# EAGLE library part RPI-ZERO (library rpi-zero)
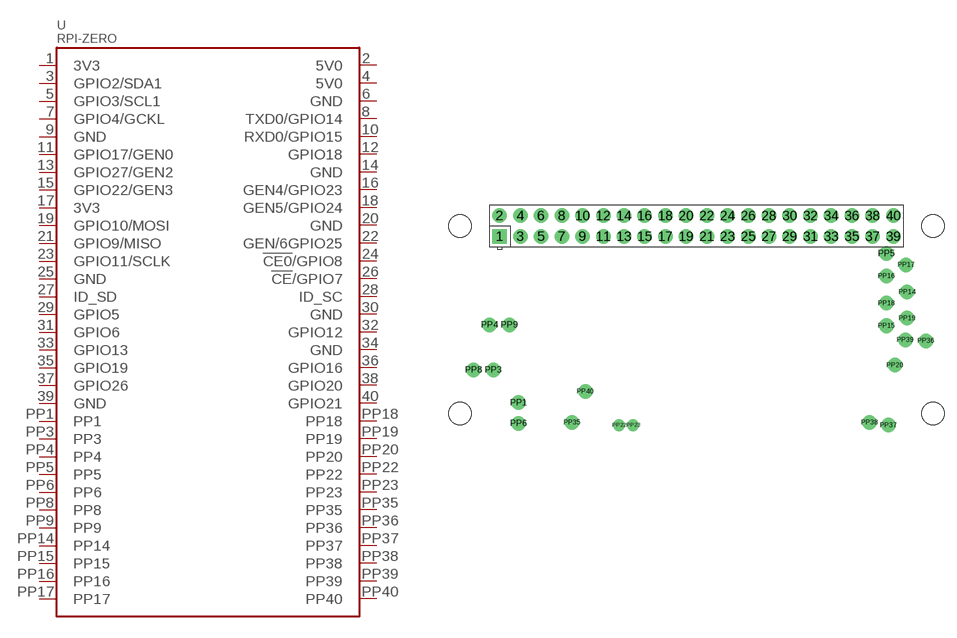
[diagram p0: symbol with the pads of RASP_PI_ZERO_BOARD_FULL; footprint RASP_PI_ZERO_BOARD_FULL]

Designator prefix -

## RPI-ZERO  [RASP_PI_ZERO_BOARD_FULL]
1  3V3  sup
2  5V0  sup
3  GPIO2/SDA1
4  5V0  sup
5  GPIO3/SCL1
6  GND  sup
7  GPIO4/GCKL
8  TXD0/GPIO14
9  GND  sup
10  RXD0/GPIO15
11  GPIO17/GEN0
12  GPIO18
13  GPIO27/GEN2
14  GND  sup
15  GPIO22/GEN3
16  GEN4/GPIO23
17  3V3  sup
18  GEN5/GPIO24
19  GPIO10/MOSI
20  GND  sup
21  GPIO9/MISO
22  GEN/6GPIO25
23  GPIO11/SCLK
24  !CE0!/GPIO8
25  GND  sup
26  !CE!/GPIO7
27  ID_SD
28  ID_SC
29  GPIO5
30  GND  sup
31  GPIO6
32  GPIO12
33  GPIO13
34  GND  sup
35  GPIO19
36  GPIO16
37  GPIO26
38  GPIO20
39  GND  sup
40  GPIO21
PP1  PP1
PP3  PP3
PP4  PP4
PP5  PP5
PP6  PP6
PP8  PP8
PP9  PP9
PP14  PP14
PP15  PP15
PP16  PP16
PP17  PP17
PP18  PP18
PP19  PP19
PP20  PP20  oc
PP22  PP22
PP23  PP23
PP35  PP35
PP36  PP36
PP37  PP37
PP38  PP38
PP39  PP39
PP40  PP40

## Footprint RASP_PI_ZERO_BOARD_FULL (pad centres in mm)
Raspberry Pi board model B+, full outline with position of big connectors & drill holes
drill 1 pad 1.778 square: 1 8.37,25.23
drill 1 pad 1.778: 2 8.37,27.77; 3 10.91,25.23; 4 10.91,27.77; 5 13.45,25.23; 6 13.45,27.77; 7 15.99,25.23; 8 15.99,27.77; 9 18.53,25.23; 10 18.53,27.77; 11 21.07,25.23; 12 21.07,27.77; 13 23.61,25.23; 14 23.61,27.77; 15 26.15,25.23; 16 26.15,27.77; 17 28.69,25.23; 18 28.69,27.77; 19 31.23,25.23; 20 31.23,27.77; 21 33.77,25.23; 22 33.77,27.77; 23 36.31,25.23; 24 36.31,27.77; 25 38.85,25.23; 26 38.85,27.77; 27 41.39,25.23; 28 41.39,27.77; 29 43.93,25.23; 30 43.93,27.77; 31 46.47,25.23; 32 46.47,27.77; 33 49.01,25.23; 34 49.01,27.77; 35 51.55,25.23; 36 51.55,27.77; 37 54.09,25.23; 38 54.09,27.77; 39 56.63,25.23; 40 56.63,27.77
drill 0.8 pad 1.778: PP1 10.699,4.832; PP3 7.593,8.858; PP4 7.133,14.38; PP5 55.796,23.124; PP6 10.699,2.301; PP8 5.177,8.858; PP9 9.549,14.38; PP14 58.327,18.407; PP15 55.796,14.265; PP16 55.796,20.363; PP17 58.212,21.743; PP18 55.796,17.027; PP19 58.327,15.186; PP20 56.832,9.434; PP35 17.257,2.416; PP36 60.628,12.425; PP37 56.026,2.071; PP38 53.726,2.416; PP39 58.097,12.54; PP40 18.867,6.212
drill 0.8 pad 1.422: PP22 23.009,2.071; PP23 24.734,2.071
hole 2.75 at 3.5,3.5
hole 2.75 at 3.5,26.5
hole 2.75 at 61.5,3.5
hole 2.75 at 61.5,26.5

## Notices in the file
Konrad Meyer (c) 2011
